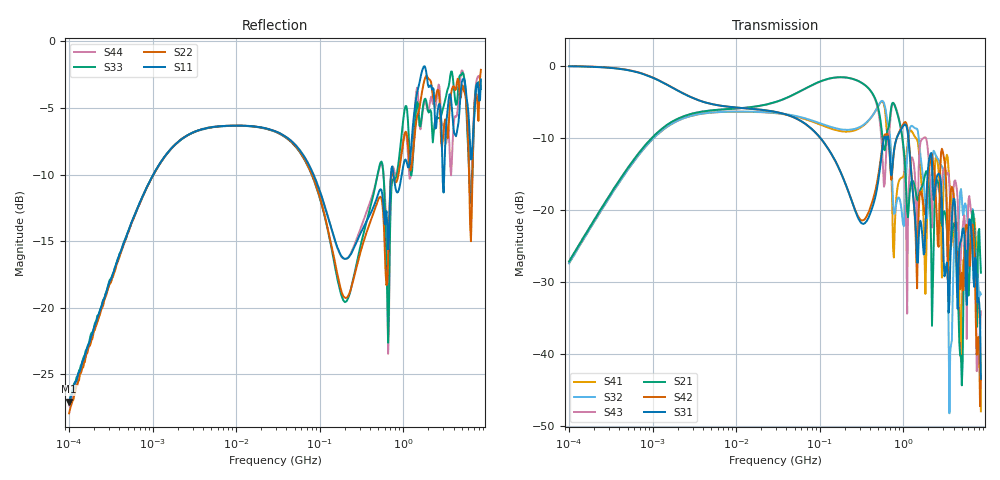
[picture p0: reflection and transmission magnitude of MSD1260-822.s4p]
# MHz S MA R 50
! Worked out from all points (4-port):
!   498 points, 100 kHz to 8.5 GHz, reference 50 ohm
!   strongest paths, dB at 100 kHz, 1.698 MHz, 29.49 MHz, 500.7 MHz, 8.5 GHz:
!     S31: -0.1, -3.0, -6.4, -16.1, -43.5
!     S42: -0.1, -3.0, -6.4, -15.4, -43.0
!     S21: -27.2, -7.8, -5.1, -5.9, -28.7
!     S43: -27.2, -7.8, -5.1, -6.2, -34.1
!     S32: -27.4, -8.1, -6.6, -5.6, -31.7
!     S41: -27.4, -8.1, -6.6, -5.6, -48.0
!   lowest |S11| = -27.1 dB at 100 kHz (marker M1), VSWR 1.09, Z = 50.3 + j4.45 ohm
!   |S11| at or under -10 dB: 84.09 MHz to 712.9 MHz (628.8 MHz wide, 158 % of centre); 766 MHz to 960.2 MHz (194.1 MHz wide, 22.5 % of centre); 2.96 GHz to 3.094 GHz (134 MHz wide, 4.43 % of centre)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
0.1  0.0444 83.8  0.04373 83.3  0.9894 -2.6  0.04263 -96.4
     0.04373 83.3  0.04016 85.6  0.04242 -95.8  0.9916 -2.5
     0.9894 -2.6  0.04242 -95.8  0.04366 84.1  0.04371 83.0
     0.04263 -96.4  0.9916 -2.5  0.04371 83.0  0.04299 85.5
127.1871  0.2166 -46.9  0.8113 -13.8  0.2632 -92.4  0.3706 84.4
          0.8113 -13.8  0.1934 -56.8  0.3804 78.1  0.2632 -92.2
          0.2632 -92.4  0.3804 78.1  0.1907 -56.4  0.8092 -13.6
          0.3706 84.4  0.2632 -92.2  0.8092 -13.6  0.2171 -46.7
561.2231  0.2674 -63.1  0.3264 -119.1  0.2659 35.8  0.565 -64.0
          0.3264 -119.1  0.247 -64.7  0.57 -64.4  0.2746 32.6
          0.2659 35.8  0.57 -64.4  0.3472 -69.3  0.2461 -132.5
          0.565 -64.0  0.2746 32.6  0.2461 -132.5  0.3432 -72.2
2062.915  0.6762 -173.2  0.1245 65.8  0.2304 165.4  0.1337 160.5
          0.1245 65.8  0.7195 -170.2  0.1308 158.5  0.2004 162.3
          0.2304 165.4  0.1308 158.5  0.5462 -165.2  0.1838 94.2
          0.1337 160.5  0.2004 162.3  0.1838 94.2  0.5765 -160.9
3651.237  0.6329 -0.6  0.05219 -84.1  0.04137 82.7  0.137 -45.9
          0.05219 -84.1  0.5983 9.6  0.01036 -1.7  0.1233 -3.4
          0.04137 82.7  0.01036 -1.7  0.7412 10.8  0.1035 -112.2
          0.137 -45.9  0.1233 -3.4  0.1035 -112.2  0.3414 -8.4
6920.76  0.4727 24.9  0.09367 -4.3  0.03333 6.1  0.08213 52.2
         0.09367 -4.3  0.4527 19.5  0.09315 8.2  0.06836 -16.8
         0.03333 6.1  0.09315 8.2  0.4402 23.1  0.08532 -60.1
         0.08213 52.2  0.06836 -16.8  0.08532 -60.1  0.4845 40.1
8500  0.7199 -38.6  0.03658 -126.2  0.006704 -150.1  0.003991 13.7
      0.03658 -126.2  0.7824 -44.0  0.02588 -151.3  0.007075 -30.5
      0.006704 -150.1  0.02588 -151.3  0.6624 -51.8  0.01973 -28.3
      0.003991 13.7  0.007075 -30.5  0.01973 -28.3  0.675 -55.5
